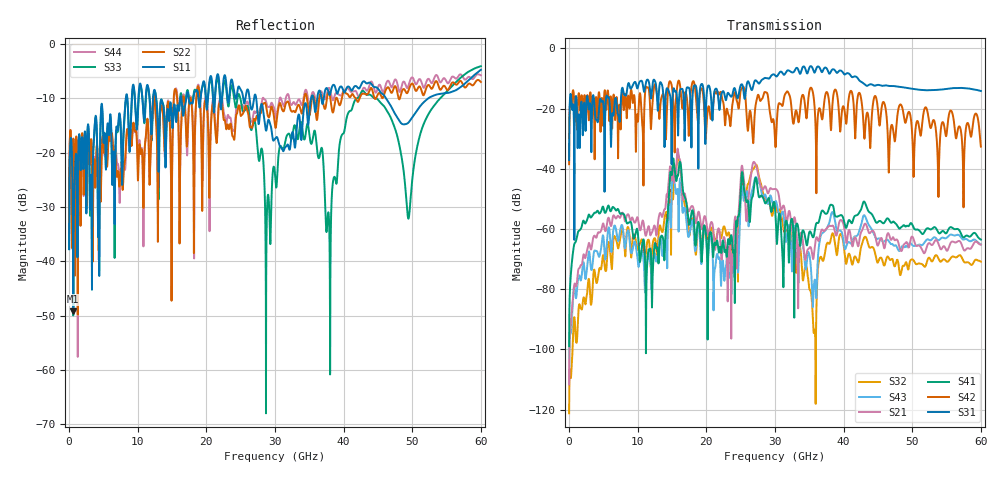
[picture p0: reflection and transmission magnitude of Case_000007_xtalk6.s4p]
! Info: Touchstone file created by circ.  Input file=CasetestDOE_NRZ_template_000007.circ
# Hz S RI R 50
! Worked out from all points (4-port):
!   6000 points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, 10 MHz to 60 GHz, reference 50 ohm
!   strongest paths, dB at 10 MHz, 15.01 GHz, 30.01 GHz, 45.01 GHz, 60 GHz:
!     S31: -37.1, -21.3, -9.0, -12.1, -14.1
!     S42: -38.5, -13.1, -30.5, -20.6, -32.6
!     S41: -99.0, -41.6, -52.9, -57.7, -63.5
!     S21: -111.6, -41.8, -46.7, -65.5, -65.2
!     S43: -111.6, -45.0, -51.2, -63.2, -65.1
!     S32: -121.3, -48.1, -51.7, -71.1, -70.9
!   lowest |S11| = -49.2 dB at 610 MHz (marker M1), VSWR 1.01, Z = 50.3 - j0.164 ohm
!   |S11| at or under -10 dB: start of sweep to 8.269 GHz; 27.26 GHz to 35.27 GHz (8.002 GHz wide, 25.6 % of centre); 46.17 GHz to 52.33 GHz (6.154 GHz wide, 12.5 % of centre)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
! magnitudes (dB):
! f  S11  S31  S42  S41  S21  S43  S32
! 10 MHz  -37.8  -37.1  -38.5  -99.0  -111.6  -111.6  -121.3
! 610 MHz  -49.2  -18.9  -13.9  -67.1  -81.8  -81.7  -93.4
! 15.88 GHz  -11.5  -28.7  -11.1  -42.1  -34.1  -49.7  -35.2
! 23.37 GHz  -9.3  -15.4  -23.4  -65.1  -65.5  -75.7  -61.9
! 26.99 GHz  -9.7  -11.0  -24.1  -45.2  -37.8  -43.9  -39.6
! 35.28 GHz  -9.9  -5.9  -13.1  -61.4  -66.6  -74.3  -81.6
! 60 GHz  -4.7  -14.1  -32.6  -63.5  -65.2  -65.1  -70.9
